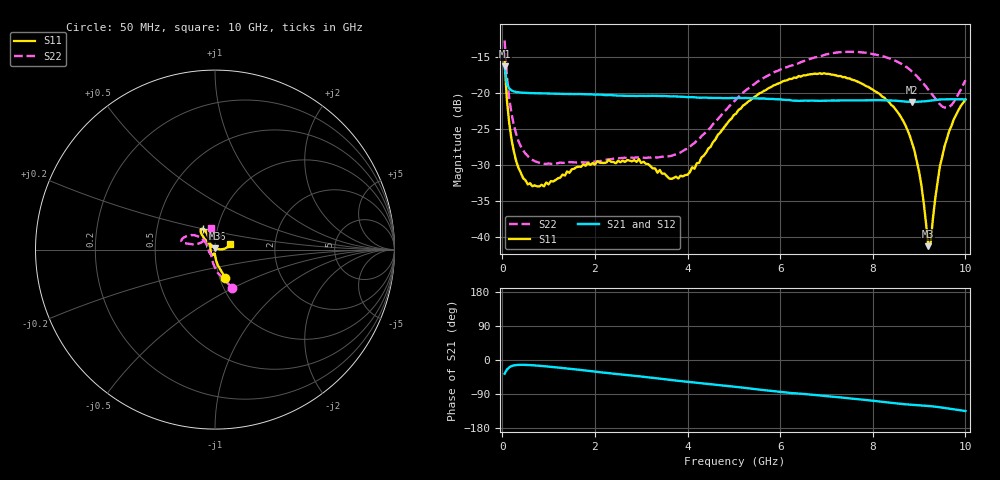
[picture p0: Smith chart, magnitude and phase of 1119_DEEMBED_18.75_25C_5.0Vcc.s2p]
!Hittite Microwave Corp.
!Digital Attenuator/PhaseShifter Rev 1.4.0
!Filename: C:\DATA\DATA\1119_DEEMBED_18.75_25C_5.0Vcc.s2p
!VNA ID: Agilent Technologies,N5224A,MY51441122,A.10.45.03
!Device type:
!2 Port Calibration.
!Temp(C): 25
!Lot Number:
!Serial Number:
!Operator:
!Misc:
!Attenuator:  18.750
# GHZ S DB R 50.0
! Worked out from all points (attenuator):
!   200 points, 50 MHz to 10 GHz, reference 50 ohm
!   highest |S21| = -16.27 dB at 50 MHz (marker M1); lowest = -21.2 dB at 8.85 GHz (marker M2)
!   lowest |S11| = -41.3 dB at 9.2 GHz (marker M3), VSWR 1.02, Z = 50.1 + j0.849 ohm
!   |S11| at or under -10 dB: start of sweep to end of sweep
!   |S22| runs from -29.9 to -12.7 dB; largest |S21 - S12| = 0.00027
!   S11 on the Smith chart (normalised r, x): 50 MHz: 1.06, -0.34; 6.6 GHz: 0.85, +0.20; 10 GHz: 1.18, +0.07
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0.05  -15.63 -70.1  -16.27 -36.2  -16.28 -36.2  -12.67 -65.8
0.1  -21.03 -79.8  -18.70 -25.3  -18.70 -25.2  -17.61 -83.0
0.2  -26.49 -86.2  -19.63 -16.1  -19.64 -16.1  -22.89 -99.7
0.35  -30.43 -90.0  -19.89 -12.9  -19.89 -12.9  -26.69 -113.7
0.55  -32.72 -95.5  -19.99 -13.1  -19.98 -13.1  -28.77 -125.2
1.75  -29.94 -120.2  -20.16 -27.1  -20.15 -27.1  -29.64 -138.8
2.95  -29.19 -132.6  -20.38 -42.9  -20.39 -42.9  -28.98 -157.7
3.4  -30.71 -154.3  -20.41 -49.1  -20.41 -49.2  -28.92 -171.1
4  -31.37 156.3  -20.56 -57.6  -20.57 -57.7  -27.75 164.7
5.05  -22.85 118.0  -20.68 -71.0  -20.70 -71.0  -20.85 140.1
5.85  -18.96 117.6  -20.82 -82.2  -20.83 -82.2  -17.14 145.1
6.6  -17.43 121.2  -21.06 -90.5  -21.08 -90.6  -15.34 153.8
6.7  -17.36 122.0  -21.05 -91.7  -21.06 -91.7  -15.12 154.8
7.5  -17.96 129.1  -21.02 -101.3  -21.03 -101.3  -14.25 164.0
8.35  -21.22 133.6  -21.03 -112.3  -21.03 -112.3  -15.14 167.9
8.85  -26.97 134.2  -21.24 -118.1  -21.24 -118.1  -17.02 167.4
9.05  -32.86 129.4  -21.19 -119.8  -21.20 -119.8  -18.33 166.4
9.2  -41.32 80.2  -21.09 -121.3  -21.10 -121.3  -19.53 163.5
9.25  -40.83 45.1  -21.05 -121.8  -21.07 -121.9  -19.94 161.7
9.35  -34.62 9.0  -20.98 -123.2  -20.99 -123.2  -20.77 156.6
9.55  -27.41 2.3  -20.86 -126.6  -20.88 -126.6  -22.01 138.5
10  -20.91 19.7  -20.88 -134.6  -20.89 -134.6  -18.21 99.8
